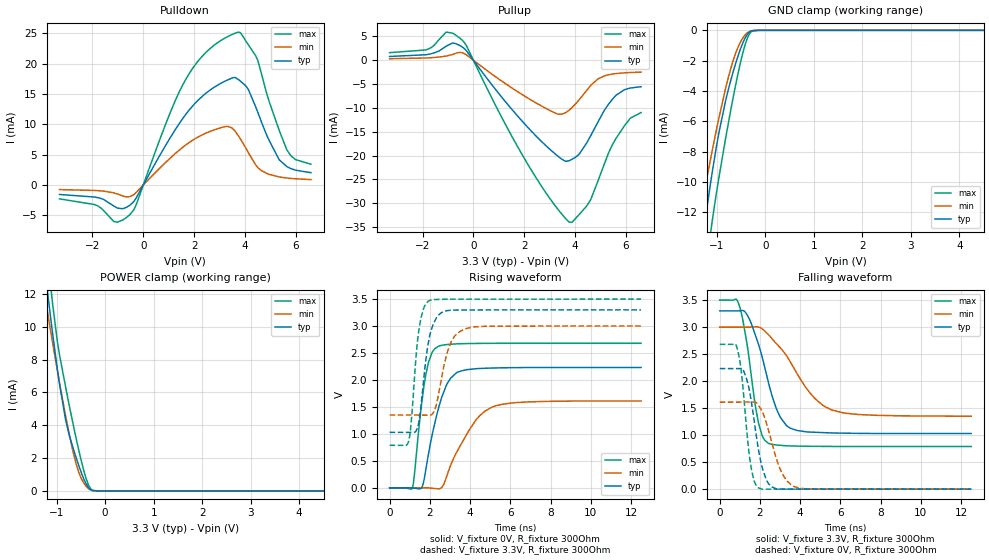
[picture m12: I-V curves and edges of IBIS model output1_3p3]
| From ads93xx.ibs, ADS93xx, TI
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|   output1_3p3 Model
[Model]   output1_3p3
Model_type   3-state
Polarity   Non-Inverting
Vmeas = 1.65
Vref = 0
Cref = 2pF
Rref = 100000
|   typ   min   max
C_comp   0.672419pF   0.55162pF   0.700875pF
[Voltage Range]   3.3   3   3.5
[Temperature Range]   27   125   -40
[Pullup Reference]   3.3   3   3.5
[Pulldown Reference]   0   0   0
[Power Clamp Reference]   3.3   3   3.5
[GND Clamp Reference]   0   0   0
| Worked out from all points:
|   slope of the pulldown table from 0 to 0.495 V, typ, clamps not added: 132 ohm
|   slope of the pullup table from 0 to 0.495 V, typ, clamps not added: 140 ohm
|   GND clamp passes 1 mA (typ) near -0.49 V on its own axis
|   POWER clamp passes 1 mA (typ) near -0.48 V on its own axis
|   falling waveform, V_fixture 3.3V, R_fixture 300Ohm: 20-80 % time 1.05ns typ, 1.86ns min, 643ps max; typ from 3.3 V to 1.03 V
|   rising waveform, V_fixture 0V, R_fixture 300Ohm: 20-80 % time 851ps typ, 1.42ns min, 518ps max; typ from 0 V to 2.23 V
|   rising waveform, V_fixture 3.3V, R_fixture 300Ohm: 20-80 % time 459ps typ, 614ps min, 369ps max; typ from 1.03 V to 3.3 V
|   falling waveform, V_fixture 0V, R_fixture 300Ohm: 20-80 % time 586ps typ, 800ps min, 424ps max; typ from 2.23 V to 0 V
[Pulldown]
|   Voltage   I(typ)   I(min)   I(max)
-3.3V     -1.567mA   -756.5uA   -2.291mA
-1.904V   -1.997mA   -906.5uA   -3.252mA
-1.162V   -3.468mA   -1.296mA   -6.029mA
-537.9mV  -3.367mA   -1.924mA   -4.923mA
1.68V     11.68mA    6.621mA    17.48mA
3.204V    17.1mA     9.611mA    24.21mA
3.739V    17.41mA    8.143mA    25.21mA
4.125V    15.82mA    5.418mA    23.2mA
4.501V    12.07mA    2.922mA    20.62mA
5.343V    4.224mA    1.339mA    9.114mA
5.66V     3.018mA    1.147mA    5.74mA
6.6V      2.03mA     885.7uA    3.418mA
[GND Clamp]
|   Voltage   I(typ)   I(min)   I(max)
-3.3V     -65.43mA   -48.13mA   -88mA
-1.419V   -16.72mA   -13.4mA    -21.78mA
-1.34V    -14.82mA   -12.03mA   -19.27mA
-1.251V   -12.75mA   -10.51mA   -16.6mA
-1.122V   -9.915mA   -8.368mA   -13.21mA
-1.092V   -9.299mA   -7.887mA   -12.52mA
-953.7mV  -6.687mA   -5.727mA   -9.638mA
-815.1mV  -4.579mA   -3.766mA   -7.051mA
-676.5mV  -2.877mA   -2.123mA   -4.639mA
-458.7mV  -789uA     -478.5uA   -1.416mA
-310.2mV  -80.27uA   -56.11uA   -160.2uA
6.6V      0A         0A         0A
[Pullup]
|   Voltage   I(typ)   I(min)   I(max)
-3.3V     793.9uA    316.8uA    1.589mA
-1.855V   1.168mA    476.1uA    2.193mA
-1.073V   2.956mA    871.8uA    5.906mA
-478.5mV  2.918mA    1.617mA    4.385mA
2.095V    -13.81mA   -7.783mA   -21.4mA
3.293V    -19.97mA   -11.24mA   -31.04mA
3.779V    -21.05mA   -10.43mA   -33.97mA
4.165V    -19.68mA   -8.29mA    -32.35mA
4.62V     -15.81mA   -5.283mA   -29.2mA
5.57V     -7.603mA   -2.824mA   -16.79mA
6.184V    -5.819mA   -2.571mA   -12.13mA
6.6V      -5.551mA   -2.496mA   -10.97mA
[POWER Clamp]
|   Voltage   I(typ)   I(min)   I(max)
-3.3V     74.57mA    53.89mA    103mA
-1.241V   13.49mA    11.88mA    16.28mA
-1.171V   11.74mA    10.61mA    14mA
-1.102V   10.06mA    9.373mA    11.94mA
-983.4mV  7.392mA    7.311mA    9.076mA
-815.1mV  4.344mA    4.58mA     6.342mA
-755.7mV  3.594mA    3.689mA    5.454mA
-656.7mV  2.576mA    2.339mA    4.022mA
-537.9mV  1.498mA    1.095mA    2.414mA
-399.3mV  475.5uA    314.3uA    830.4uA
-300.3mV  81.22uA    66.3uA     149.3uA
6.6V      0A         0A         0A
[Ramp]
R_load = 300
|   typ   min   max
dV/dt_r   1.33886/8.50519e-10   0.966313/1.42268e-09   1.6082/5.17415e-10
dV/dt_f   1.36266/1.04898e-09   0.990485/1.854e-09   1.62645/6.42114e-10
[Falling Waveform]
V_fixture = 3.3V
V_fixture_min = 3V
V_fixture_max = 3.5V
R_fixture = 300Ohm
C_fixture = 0F
|   Time   V(typ)   V(min)   V(max)
0s        3.3V       3V         3.5V
946.7ps   3.299V     3V         3.427V
1.357ns   3.23V      3V         2.685V
1.929ns   2.677V     2.999V     1.222V
2.421ns   1.973V     2.86V      847.4mV
2.887ns   1.427V     2.665V     813.6mV
3.391ns   1.155V     2.428V     801mV
4.488ns   1.056V     1.779V     792.9mV
5.57ns    1.04V      1.466V     790.2mV
12.5ns    1.029V     1.349V     789.3mV
[Rising Waveform]
V_fixture = 0V
V_fixture_min = 0V
V_fixture_max = 0V
R_fixture = 300Ohm
C_fixture = 0F
|   Time   V(typ)   V(min)   V(max)
0s        231.6nV    18.3uV     -199.4nV
1.144ns   74.63uV    180uV      13.71mV
1.582ns   -3.569mV   241.9uV    1.528V
1.795ns   323.7mV    271.9uV    2.088V
2.1ns     952.6mV    -6.306mV   2.504V
2.421ns   1.462V     -18.23mV   2.625V
3.317ns   2.131V     648.7mV    2.669V
4.327ns   2.21V      1.274V     2.677V
5.112ns   2.221V     1.5V       2.68V
12.5ns    2.231V     1.611V     2.68V
[Rising Waveform]
V_fixture = 3.3V
V_fixture_min = 3V
V_fixture_max = 3.5V
R_fixture = 300Ohm
C_fixture = 0F
|   Time   V(typ)   V(min)   V(max)
0s        1.029V     1.349V     789.3mV
946.7ps   1.028V     1.349V     862mV
1.057ns   1.028V     1.349V     1.15V
1.455ns   1.222V     1.349V     2.926V
1.687ns   1.978V     1.349V     3.322V
1.929ns   2.696V     1.348V     3.463V
2.277ns   3.114V     1.48V      3.492V
3.006ns   3.291V     2.661V     3.498V
3.692ns   3.297V     2.937V     3.498V
12.5ns    3.3V       3V         3.5V
[Falling Waveform]
|Gnd
V_fixture = 0V
V_fixture_min = 0V
V_fixture_max = 0V
R_fixture = 300Ohm
C_fixture = 0F
|   Time   V(typ)   V(min)   V(max)
0s        2.231V     1.61V      2.68V
873.2ps   2.231V     1.611V     2.596V
1.036ns   2.233V     1.611V     2.284V
1.185ns   2.192V     1.611V     1.76V
1.568ns   1.625V     1.612V     384.6mV
1.929ns   724mV      1.549V     21.82mV
2.439ns   93.95mV    1.071V     -734.8uV
3.083ns   1.874mV    306.1mV    -687.7uV
3.771ns   1.737mV    37.89mV    -637.5uV
12.5ns    379nV      15.76uV    -80.95nV
